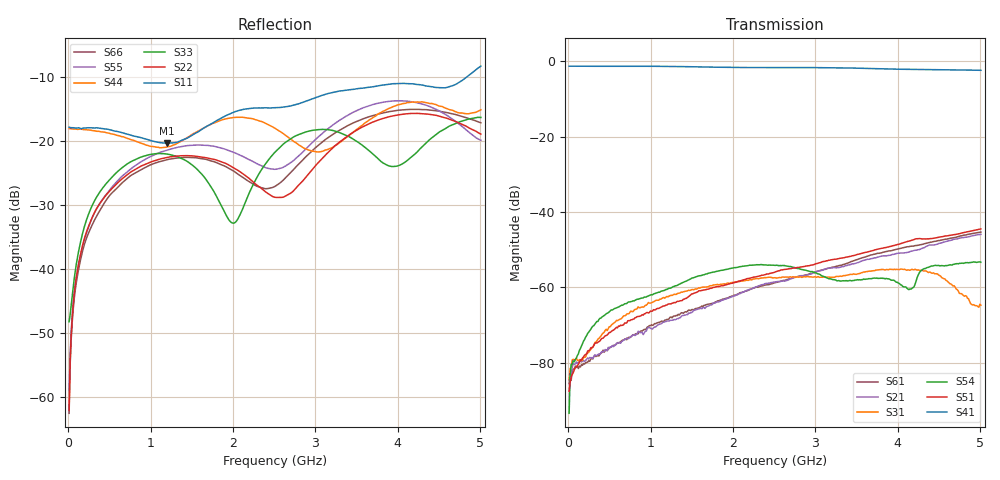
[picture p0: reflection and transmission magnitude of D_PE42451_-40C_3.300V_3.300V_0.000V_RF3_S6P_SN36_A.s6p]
! Device ID: PE42451
! Serial: 36
! Insertion: A
! Temp: -40C
! VDD: 3.300
! Control_Hi: 100.000
! Control_Lo: 0.000
! Logic State: RF3
! Port 1: RFC
! Port 2: RF1
! Port 3: RF2
! Port 4: RF3
! Port 5: RF4
! Port 6: RF5
! V1 = 3.30
! V2 = 3.30
! V3 = 0.00
! V4 = 0.00
! IDD: 1.604920e-05
#  Hz  S  RI  R  50
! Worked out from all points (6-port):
!   401 points, 10 MHz to 5.01 GHz, reference 50 ohm
!   strongest paths, dB at 10 MHz, 1.26 GHz, 2.51 GHz, 3.76 GHz, 5.01 GHz:
!     S41: -1.3, -1.3, -1.6, -1.9, -2.4
!     S51: -87.6, -64.3, -56.0, -49.9, -44.5
!     S54: -93.5, -60.0, -54.2, -57.6, -53.4
!     S31: -84.5, -62.2, -57.5, -55.4, -64.8
!     S21: -84.7, -68.8, -58.6, -52.0, -46.0
!     S61: -85.6, -68.1, -58.8, -51.0, -45.3
!   lowest |S11| = -20.3 dB at 1.198 GHz (marker M1), VSWR 1.21, Z = 55.4 - j8.62 ohm
!   |S11| at or under -10 dB: start of sweep to 4.836 GHz
